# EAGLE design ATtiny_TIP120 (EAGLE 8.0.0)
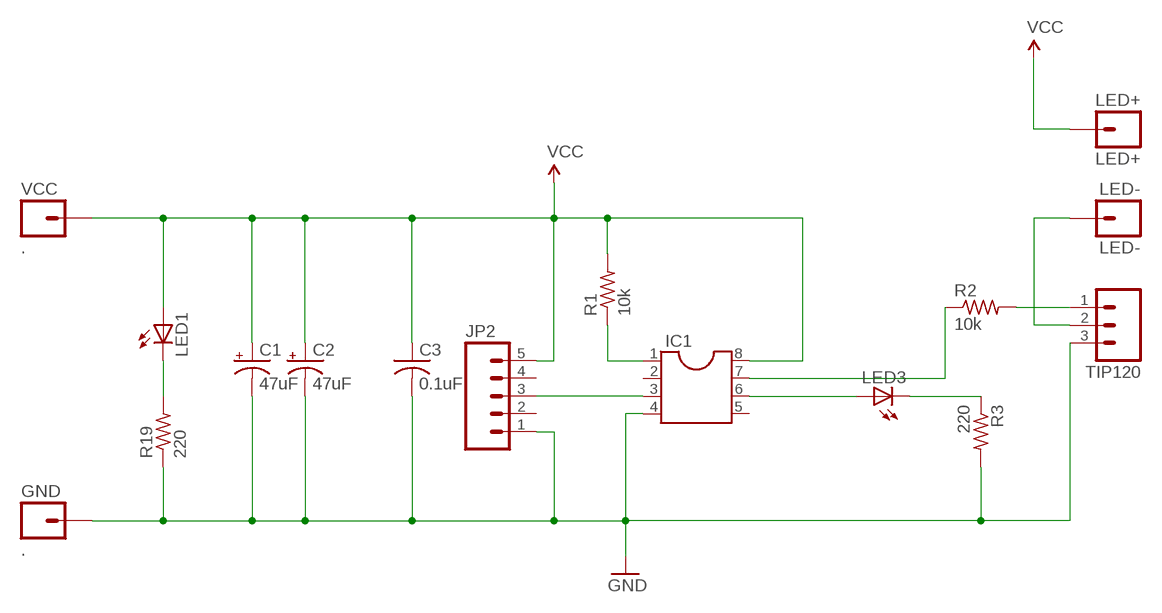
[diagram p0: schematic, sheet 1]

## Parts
C1  47uF  CAP_POLPTH4  [CPOL-RADIAL-1000UF-25V]
C2  47uF  CAP_POLPTH4  [CPOL-RADIAL-1000UF-25V]
C3  0.1uF  C-US025-025X050  [C025-025X050]
GND  .  M01OFFSET  [1X01_OFFSET]
IC1  DIL8S  [SOCKET-08]
JP2  M05LOCK_LONGPADS  [1X05_LOCK_LONGPADS]
LED1  LED5MM  [LED5MM]
LED3  LED5MM  [LED5MM]
LED+  LED+  M01OFFSET  [1X01_OFFSET]
LED-  LED-  M01OFFSET  [1X01_OFFSET]
R1  10k  R-US_0207/7  [0207/7]
R2  10k  R-US_0207/7  [0207/7]
R3  220  R-US_0207/7  [0207/7]
R19  220  R-US_0207/7  [0207/7]
TIP120  M03LOCK_LONGPADS  [1X03_LOCK_LONGPADS]
VCC  .  M01OFFSET  [1X01_OFFSET]

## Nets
GND: C1.2(-) C2.2(-) C3.2 GND.1 IC1.4 JP2.1 R3.2 R19.1 TIP120.3
N$1: IC1.1 R1.1
N$2: IC1.7 R2.1
N$3: IC1.3 JP2.3
N$4: R2.2 TIP120.1
N$6: LED1.K(C) R19.2
N$7: LED3.K(C) R3.1
N$8: LED-.1 TIP120.2
N$10: IC1.6 LED3.A
VCC: C1.1(+) C2.1(+) C3.1 IC1.8 JP2.5 LED1.A LED+.1 R1.2 VCC.1
Unconnected: IC1.2 IC1.5 JP2.2 JP2.4

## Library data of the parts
C1 C2 = SparkFun:CAP_POL: Capacitor Polarized
C3 = adafruit-2014:C-US: CAPACITOR, American symbol
GND LED+ LED- VCC = SparkFun:M01: Header 1
IC1 = ic-package:DIL8: Dual In Line / Socket
JP2 = SparkFun:M05: Header 5 Standard 5-pin 0.1" header. Use with straight break away headers (SKU : PRT-00116), right angle break away headers (PRT-00553), swiss pins (PRT-00743), machine pins (PRT-00117), and female headers (PRT-00115). Molex polarized connector foot print use with SKU : PRT-08230 with associated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
LED1 LED3 = adafruit-2014:LED: LED
R1-R3 R19 = adafruit-2014:R-US_: RESISTOR, American symbol
TIP120 = SparkFun:M03: Header 3 Standard 3-pin 0.1" header. Use with straight break away headers (SKU : PRT-00116), right angle break away headers (PRT-00553), swiss pins (PRT-00743), machine pins (PRT-00117), and female headers (PRT-00115). Molex polarized connector foot print use with SKU : PRT-08232 with associated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

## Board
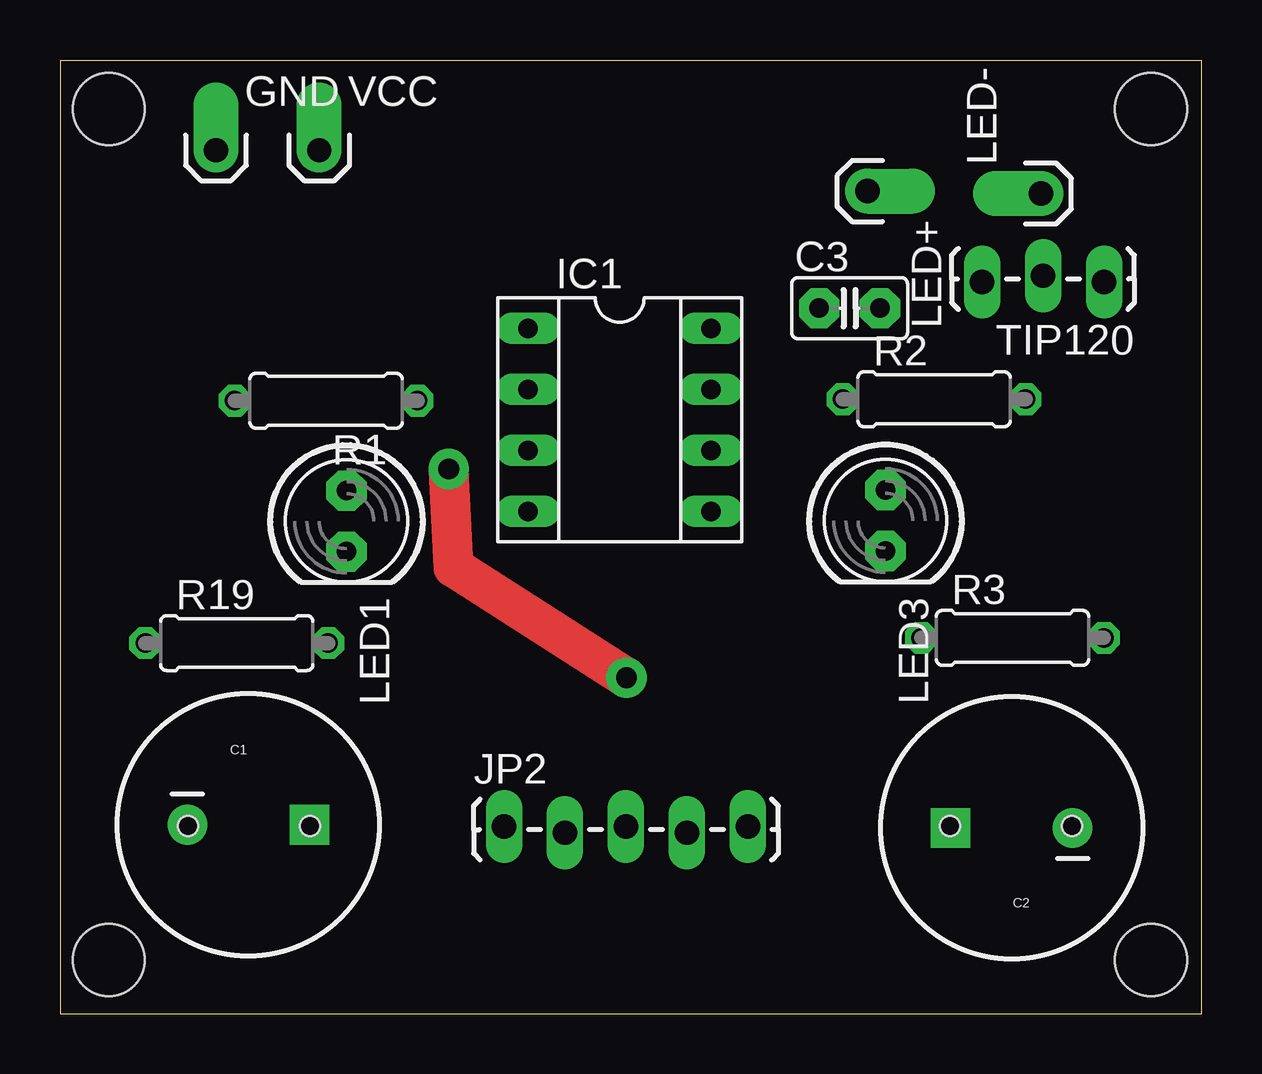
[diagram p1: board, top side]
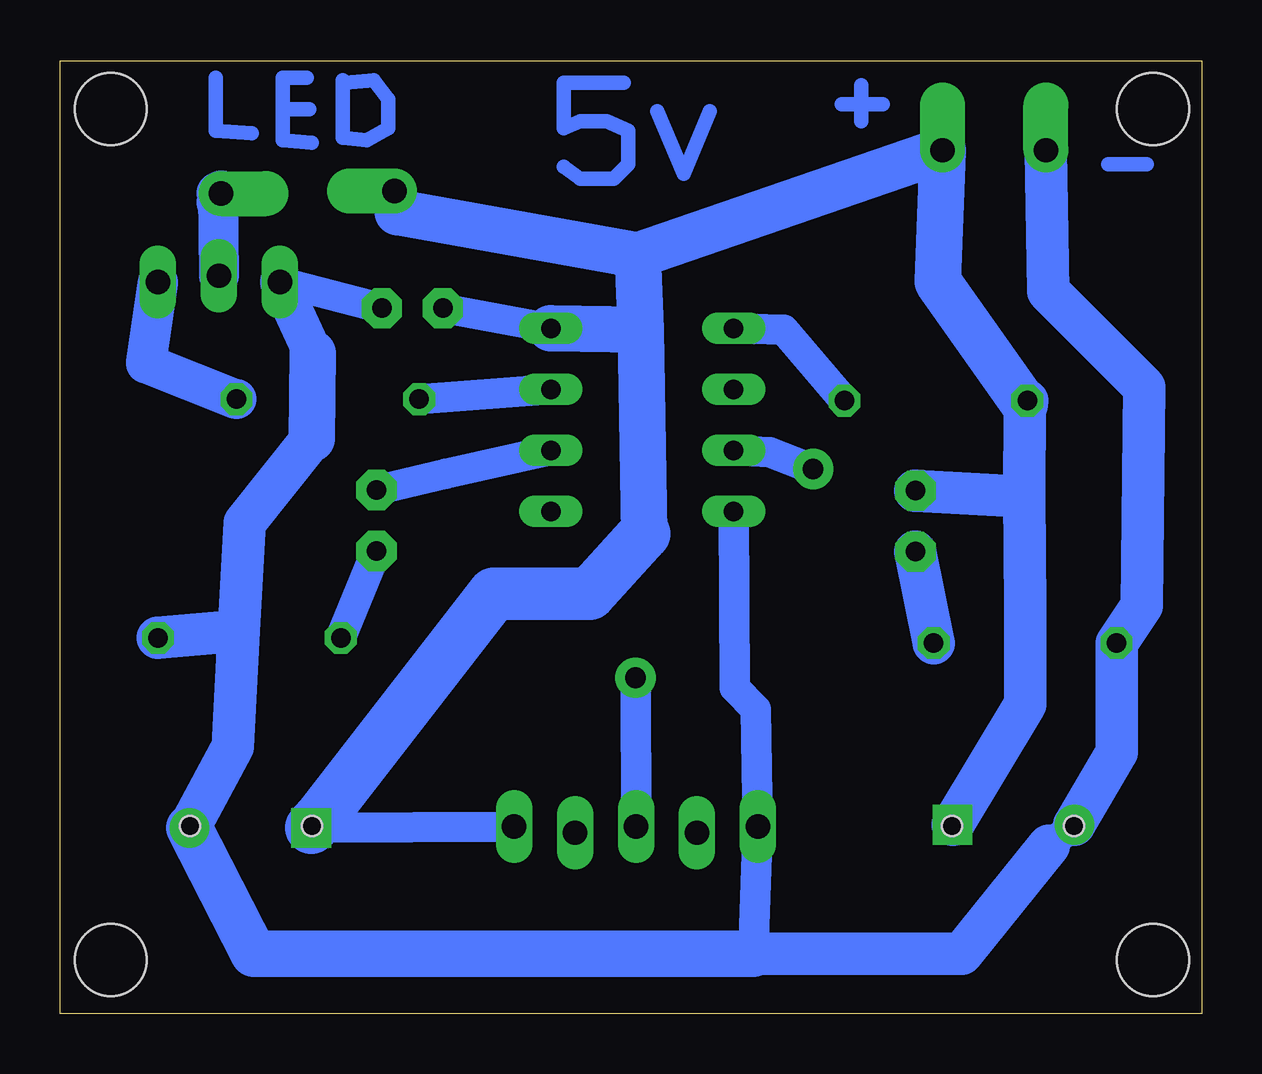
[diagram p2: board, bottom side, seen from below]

Size 47.58 x 39.71 mm. Coordinates in mm from the lower left corner, seen from the top.
Outline: 0,0 47.58,0 47.58,39.71 0,39.71 0,0
Copper layers (1*16): Top 0.035mm / dielectric 1.5mm / Bottom 0.035mm
Design rules "default": minimum track width 10mil, minimum drill 24mil, track to track 8mil, track to pad 8mil, pad to pad 8mil, via to via 8mil, smd to smd 8mil, copper to edge 40mil, drill to drill 8mil, minimum pad ring 10mil, minimum via ring 8mil, stop-mask expansion 4mil, vias tented up to drill 0mil, thermal gap 10mil
Holes 0.84 mm at 10.41,7.83 5.33,7.83 37.08,7.83 42.16,7.83
Holes 3 mm at 2.03,2.24 45.47,2.24 2.03,37.71 45.47,37.71

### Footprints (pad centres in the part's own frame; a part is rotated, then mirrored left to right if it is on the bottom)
CPOL-RADIAL-1000UF-25V = drill 0.7 pad 1.651 square: 1 2.54,0 | drill 0.7 pad 1.651: 2 -2.54,0
C025-025X050 = drill 0.813 pad 1.676 octagon: 1 -1.27,0; 2 1.27,0
1X01_OFFSET = drill 1.016 pad 1.88 offset: 1 0,0
SOCKET-08 = drill 0.813 long: 1 -3.81,-3.81; 2 -1.27,-3.81; 3 1.27,-3.81; 4 3.81,-3.81; 5 3.81,3.81; 6 1.27,3.81; 7 -1.27,3.81; 8 -3.81,3.81
1X05_LOCK_LONGPADS = drill 1.016 long: 1 0,0; 2 2.54,-0.254; 3 5.08,0; 4 7.62,-0.254; 5 10.16,0
LED5MM = drill 0.813 pad 1.676 octagon: A -1.27,0; K 1.27,0
0207/7 = drill 0.813 octagon: 1 -3.81,0; 2 3.81,0
1X03_LOCK_LONGPADS = drill 1.016 long: 1 0,0; 2 2.54,-0.254; 3 5.08,0

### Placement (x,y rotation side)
C1  7.85,7.88 0 top
C2  39.65,7.75 180 top
C3  32.9,29.4 0 top
GND  6.5,35.98 0 top
IC1  23.32,24.75 270 top
JP2  18.5,7.8 0 top
LED1  11.94,20.53 270 top
LED3  34.39,20.55 270 top
LED+  33.64,34.28 270 top
LED-  40.87,34.18 90 top
R1  11.09,25.55 180 top
R2  36.42,25.61 0 top
R3  39.69,15.66 0 top
R19  7.37,15.45 0 top
TIP120  43.5,30.5 180 top
VCC  10.8,35.98 0 top

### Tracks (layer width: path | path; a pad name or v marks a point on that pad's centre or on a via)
GND
  Bottom 1.27: 6.37,7.01 C1.2 | C3.2 TIP120.3 | IC1.4 19.46,13.6 18.6,12.7 JP2.1 18.7,2.5
  Bottom 1.676: TIP120.3 37.06,27.53
  Bottom 1.778: C2.2 40.39,11.13 40.13,15.96 | 40.13,15.96 39.88,20.47 37.09,23.96 | R3.2 40.13,15.96 | C1.2 3.56,10.89 R19.1 2.5,17 2.4,26.1 6.4,30.1 GND.1 | 18.7,2.5 10,2.5 6.37,7.01
  Bottom 1.93: 37.09,23.96 37.06,27.53 | 18.7,2.5 39.5,2.5 C2.2
N$1
  Bottom 1.27: IC1.1 17.42,28.5 R1.1
N$2
  Bottom 1.27: R2.1 IC1.7
N$3  (via drill 0.86 pad 1.68)
  Top 1.676: v23.6,14 16.4,18.6 v16.2,22.7
  Bottom 1.27: v16.2,22.7 18,23.4 IC1.3 | JP2.3 v23.6,14
N$4
  Bottom 1.676: TIP120.1 44,27.1 R2.2
N$5
  Bottom 0.61: 24.1,38.8 26.6,38.8 26.6,36.9 25.9,37.2 24.8,37.2 23.9,36.8 23.9,35.4 24.5,34.8 25.9,34.8 26.6,35.3
N$6
  Bottom 1.778: R19.2 LED1.K
N$7
  Bottom 1.27: LED3.K R3.1
N$8
  Bottom 1.676: 41,34.19 TIP120.2
  Bottom 1.778: 40.92,33.81 41,34.19
  Bottom 1.93: LED-.1 40.92,33.81
N$9
  Bottom 0.61: 20.5,37.6 21.6,35 22.7,37.6
N$10
  Bottom 1.27: IC1.6 31.5,22.5 LED3.A
N$11
  Bottom 0.61: 41.1,39 41.1,36.8 39.6,36.7
N$12
  Bottom 0.61: 37.1,36.3 38.3,36.4 38.3,39 37.3,39
N$13
  Bottom 0.61: 38.2,37.7 37.2,37.7
N$14
  Bottom 0.61: 35.8,38.9 35.8,36.5 34.8,36.4 33.9,36.9 33.9,38.1 34.5,38.9 35.7,38.8
N$15
  Bottom 0.61: 2.3,35.4 3.9,35.4
N$16
  Bottom 0.61: 14.2,38.7 14.2,37.2
N$17
  Bottom 0.61: 13.3,37.9 15,37.9
VCC
  Bottom 1.27: IC1.8 C3.1 | JP2.5 C2.1
  Bottom 1.778: 7.41,21.55 7.37,25.38 R1.2 | C1.1 7.37,12.91 7.37,16.99 7.41,21.55 | LED1.A 7.41,21.55 | 33.5,33.4 LED+.1
  Bottom 1.93: 23.38,28.51 23.25,20.01 | 23.38,28.51 23.5,31.6 | 23.5,31.6 VCC.1 11,30.5 7.37,25.38 | 23.5,31.6 33.5,33.4 | 23.38,28.51 IC1.8
  Bottom 2.184: C2.1 36.76,8.16 29.5,17.5 25.5,17.5 23.25,20.01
